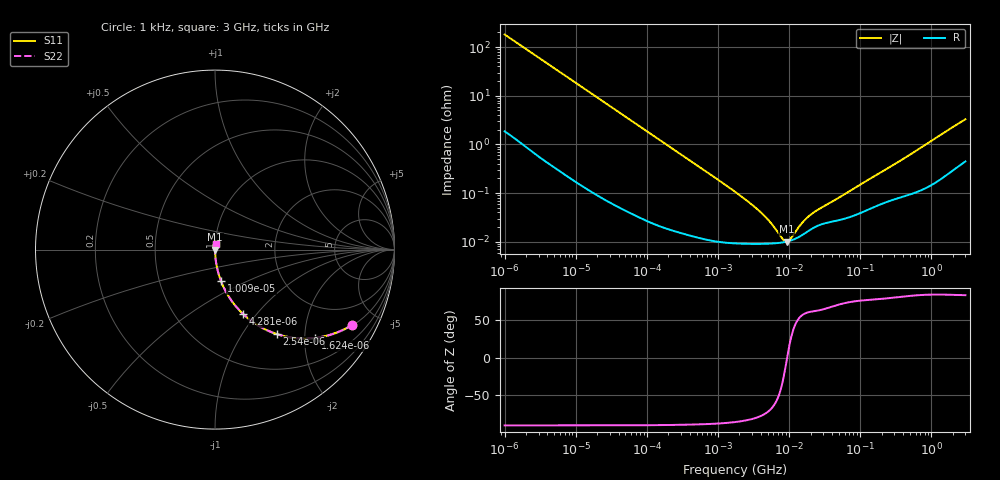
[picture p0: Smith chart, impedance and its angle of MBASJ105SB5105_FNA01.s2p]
! MBASJ105SB5105_FNA01  S-PARAMETER MODEL  ( Standard Model )
! Model Generated by TAIYO YUDEN Corporation (http://www.ty-top.com)
! Version 1.0
! TAIYO YUDEN Control No. 220601
! Copyright(c) 2013 TAIYO YUDEN CO.,LTD. All Rights Reserved.
! Product Description (link to TY-COMPAS)
! https://ds.yuden.co.jp/TYCOMPAS/or/detail?pn=MBASJ105SB5105KFNA01&u=M
! Products Name : Multilayer Ceramic Capacitors
! Characteristics :
!  Capacitance : 1 [uF] , Rated Voltage : 6.3 [V] , TCC : X5R
!  Case Size : 1.0 x 0.5 / 0.039 x 0.02 [mm/inch] , Thickness : 0.5 / 0.02 [mm/inch]
!  (Conditions: Temperature = 25 [degC] , DC Bias Voltage = 0 [V])
! External Node Assignments :
!  1  o---| |---o  2
! GND o---------o GND
! Frequency Range : 1kHz  -  3GHz  [ 401 STEP ]
# MHZ S RI R 50
! Freq[MHz].  S11 Real  S11 Imag  S21 Real  S21 Imag  S12 Real  S12 Imag  S22 Real  S22 Imag
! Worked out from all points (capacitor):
!   401 points, 1 kHz to 3 GHz, reference 50 ohm
!   read as one part in series: C = 872 nF near 1.077 kHz
!   lowest |Z| = 10.1 mohm at 9.273 MHz (marker M1)
!   series resonance near 9.368 MHz, so ESL is about 330 pH
!   S11 on the Smith chart (normalised r, x): 1 kHz: 1.04, -3.64; 1.624 kHz: 1.02, -2.25; 2.54 kHz: 1.01, -1.44; 4.281 kHz: 1.01, -0.86; 10.09 kHz: 1.00, -0.37; 3 GHz: 1.01, +0.07
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0.001  0.766 -0.4183  0.234 0.4183  0.234 0.4183  0.766 -0.4183
0.001205  0.6943 -0.4556  0.3057 0.4556  0.3057 0.4556  0.6943 -0.4556
0.001624  0.5584 -0.4917  0.4416 0.4917  0.4416 0.4917  0.5584 -0.4917
0.00254  0.3438 -0.4703  0.6562 0.4703  0.6562 0.4703  0.3438 -0.4703
0.004281  0.158 -0.3602  0.842 0.3602  0.842 0.3602  0.158 -0.3602
0.006215  0.0828 -0.2711  0.9172 0.2711  0.9172 0.2711  0.0828 -0.2711
0.010091  0.0339 -0.1765  0.9661 0.1765  0.9661 0.1765  0.0339 -0.1765
0.01216  0.0239 -0.1482  0.9761 0.1482  0.9761 0.1482  0.0239 -0.1482
0.033275  0.00369 -0.0556  0.9963 0.0556  0.9963 0.0556  0.00369 -0.0556
0.147855  0.000371 -0.0127  0.9996 0.0127  0.9996 0.0127  0.000371 -0.0127
1.732051  9.37e-05 -0.00106  0.9999 0.00106  0.9999 0.00106  9.37e-05 -0.00106
2.812335  9.07e-05 -0.000617  0.9999 0.000617  0.9999 0.000617  9.07e-05 -0.000617
4.083148  9.05e-05 -0.000379  0.9999 0.000379  0.9999 0.000379  9.05e-05 -0.000379
5.502215  9.17e-05 -0.000228  0.9999 0.000228  0.9999 0.000228  9.17e-05 -0.000228
7.988506  9.66e-05 -6.57e-05  0.9999 6.57e-05  0.9999 6.57e-05  9.66e-05 -6.57e-05
8.606987  9.84e-05 -3.48e-05  0.9999 3.48e-05  0.9999 3.48e-05  9.84e-05 -3.48e-05
9.273352  0.000101 -4.11e-06  0.9999 4.11e-06  0.9999 4.11e-06  0.000101 -4.11e-06
10.37087  0.000105 4.2e-05  0.9999 -4.2e-05  0.9999 -4.2e-05  0.000105 4.2e-05
16.22291  0.000146 0.000229  0.9999 -0.000229  0.9999 -0.000229  0.000146 0.000229
21.06097  0.000186 0.000332  0.9998 -0.000332  0.9998 -0.000332  0.000186 0.000332
256.0921  0.000696 0.00331  0.9993 -0.00331  0.9993 -0.00331  0.000696 0.00331
3000  0.0055 0.0323  0.9945 -0.0323  0.9945 -0.0323  0.0055 0.0323
